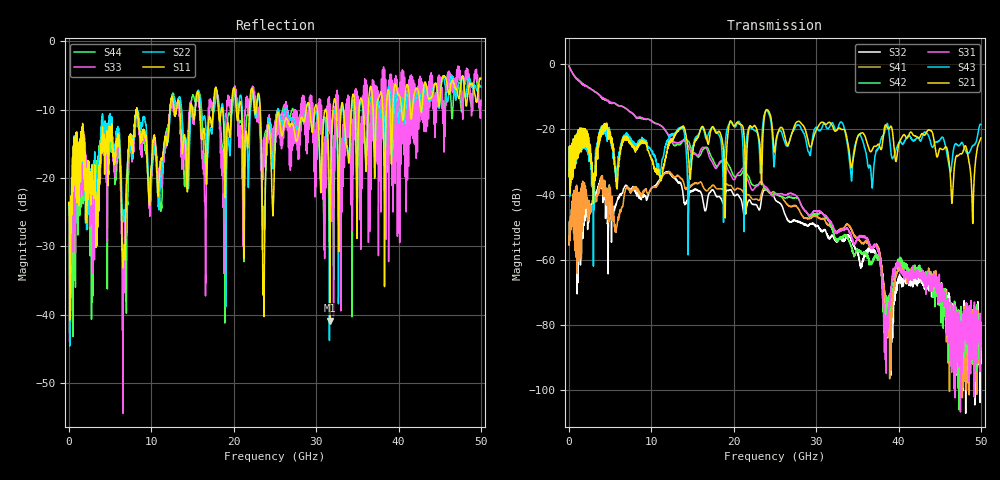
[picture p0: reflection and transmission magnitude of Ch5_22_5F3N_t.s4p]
!Agilent Technologies,N5247A,US51170199,A.09.90.13
!Agilent N5247A: A.09.90.13
!Date: Tuesday, December 08, 2015 12:51:22
!Correction: S11(Full 4 Port(1,2,3,4))
!S12(Full 4 Port(1,2,3,4))
!S13(Full 4 Port(1,2,3,4))
!S14(Full 4 Port(1,2,3,4))
!S21(Full 4 Port(1,2,3,4))
!S22(Full 4 Port(1,2,3,4))
!S23(Full 4 Port(1,2,3,4))
!S24(Full 4 Port(1,2,3,4))
!S31(Full 4 Port(1,2,3,4))
!S32(Full 4 Port(1,2,3,4))
!S33(Full 4 Port(1,2,3,4))
!S34(Full 4 Port(1,2,3,4))
!S41(Full 4 Port(1,2,3,4))
!S42(Full 4 Port(1,2,3,4))
!S43(Full 4 Port(1,2,3,4))
!S44(Full 4 Port(1,2,3,4))
!S4P File: Measurements: <S11,S12,S13,S14>,
!<S21,S22,S23,S24>,
!<S31,S32,S33,S34>,
!<S41,S42,S43,S44>:
# Hz S  dB  R 50
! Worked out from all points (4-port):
!   3201 points, 10 MHz to 50 GHz, reference 50 ohm
!   strongest paths, dB at 10 MHz, 12.51 GHz, 25 GHz, 37.5 GHz, 50 GHz:
!     S21: -34.4, -23.5, -26.2, -24.6, -22.6
!     S43: -34.5, -21.7, -27.7, -26.1, -18.5
!     S31: -0.6, -23.7, -39.7, -57.0, -85.2
!     S42: -0.6, -24.1, -39.5, -59.0, -85.4
!     S41: -55.5, -34.1, -39.7, -56.0, -84.7
!     S32: -55.3, -34.5, -41.4, -59.4, -85.4
!   lowest |S11| = -40.9 dB at 31.68 GHz (marker M1), VSWR 1.02, Z = 50 + j0.904 ohm
!   |S11| at or under -10 dB: start of sweep to 8.209 GHz; 8.248 GHz to 12.25 GHz (3.999 GHz wide, 39 % of centre); 23.22 GHz to 28.81 GHz (5.59 GHz wide, 21.5 % of centre)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
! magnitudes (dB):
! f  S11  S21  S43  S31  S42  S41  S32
! 10 MHz  -23.9  -34.4  -34.5  -0.6  -0.6  -55.5  -55.3
! 11.98 GHz  -14.4  -25.9  -23.7  -21.3  -21.6  -33.4  -33.2
! 31.68 GHz  -40.9  -17.9  -18.9  -48.0  -48.9  -49.5  -53.1
! 37.33 GHz  -9.8  -25.1  -26.6  -56.2  -58.5  -55.4  -58.9
! 38.49 GHz  -11.1  -18.7  -19.0  -78.2  -76.3  -76.4  -74.9
! 39.96 GHz  -7.8  -25.5  -24.6  -61.1  -60.8  -63.6  -66.5
! 50 GHz  -5.4  -22.6  -18.5  -85.2  -85.4  -84.7  -85.4
